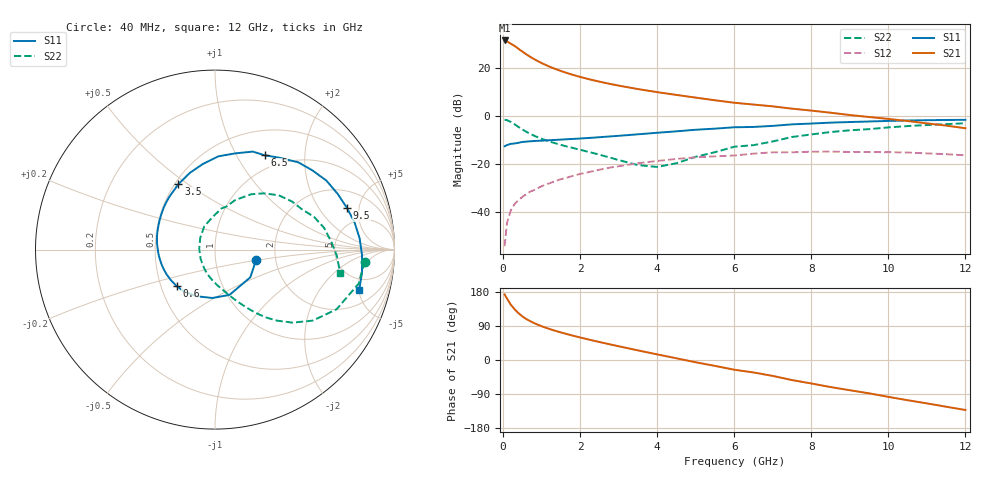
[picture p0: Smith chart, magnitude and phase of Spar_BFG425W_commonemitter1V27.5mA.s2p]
! Filename: 127bfg425.001
! BFG425W Field C1
! V1=8.847E-001V,V2=1.000E+000V, I1=4.360E-004A, I2=2.749E-002A
# GHz  S  MA  R 50
!  S11  S21  S12  S22
!Freq(GHz)  Mag  Ang  Mag  Ang  Mag  Ang  Mag  Ang
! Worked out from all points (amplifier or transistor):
!   44 points, 40 MHz to 12 GHz, reference 50 ohm
!   highest |S21| = 31.4 dB at 40 MHz (marker M1)
!   |S21| within 3 dB of that: start of sweep to 361.5 MHz
!   unconditionally stable (mu >= 1): start of sweep to 74.84 MHz; 887.2 MHz to end of sweep
!   at 700 MHz: K = 0.91, MSG = 28.0 dB, |S12| = -31.4 dB
!   at 2.4 GHz: K = 1.22, MAG = 15.8 dB, |S12| = -22.6 dB
!   at 12 GHz: K = 1.38, MAG = 1.9 dB, |S12| = -16.3 dB
!   S11 on the Smith chart (normalised r, x): 40 MHz: 1.58, -0.20; 600 MHz: 0.60, -0.27; 3.5 GHz: 0.52, +0.46; 6.5 GHz: 0.81, +1.31; 9.5 GHz: 3.27, +3.74; 12 GHz: 3.45, -5.05
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0.04  0.236 -14.8  36.96 173.0  0.002 66.7  0.837 -4.6
0.1  0.25 -38.2  35.63 162.4  0.006 79.1  0.823 -13.3
0.2  0.265 -72.2  31.58 145.9  0.011 72.4  0.755 -26.1
0.3  0.27 -93.0  28.45 133.8  0.015 67.6  0.673 -36.0
0.4  0.279 -111.2  24.83 123.6  0.018 64.5  0.594 -43.2
0.5  0.29 -125.6  21.71 115.1  0.021 62.6  0.527 -48.7
0.6  0.295 -136.5  19.12 108.4  0.024 61.4  0.474 -53.0
0.7  0.299 -145.2  16.99 102.7  0.027 60.5  0.429 -56.4
0.8  0.303 -152.8  15.24 97.6  0.029 59.9  0.393 -59.3
0.9  0.306 -159.2  13.8 93.2  0.032 59.2  0.363 -61.8
1.1  0.312 -169.9  11.53 85.5  0.038 57.7  0.317 -66.4
1.3  0.318 -178.7  9.869 78.8  0.043 56.3  0.281 -70.7
1.6  0.328 170.1  8.091 69.9  0.051 53.5  0.24 -76.8
2.2  0.35 151.6  5.891 54.6  0.068 46.5  0.182 -91.2
2.8  0.379 135.7  4.598 40.7  0.086 38.4  0.136 -110.5
3.5  0.418 119.2  3.629 25.4  0.105 28.0  0.096 -146.1
4.5  0.482 98.0  2.742 4.5  0.129 12.0  0.105 141.7
6.5  0.594 62.3  1.731 -32.9  0.166 -17.4  0.249 75.0
8.5  0.73 31.8  1.173 -71.4  0.183 -53.3  0.466 40.6
9.5  0.771 17.5  0.955 -88.0  0.179 -69.0  0.535 24.7
10.5  0.808 4.5  0.789 -106.1  0.175 -86.5  0.62 11.2
12  0.834 -15.5  0.558 -131.9  0.153 -114.0  0.709 -10.4
